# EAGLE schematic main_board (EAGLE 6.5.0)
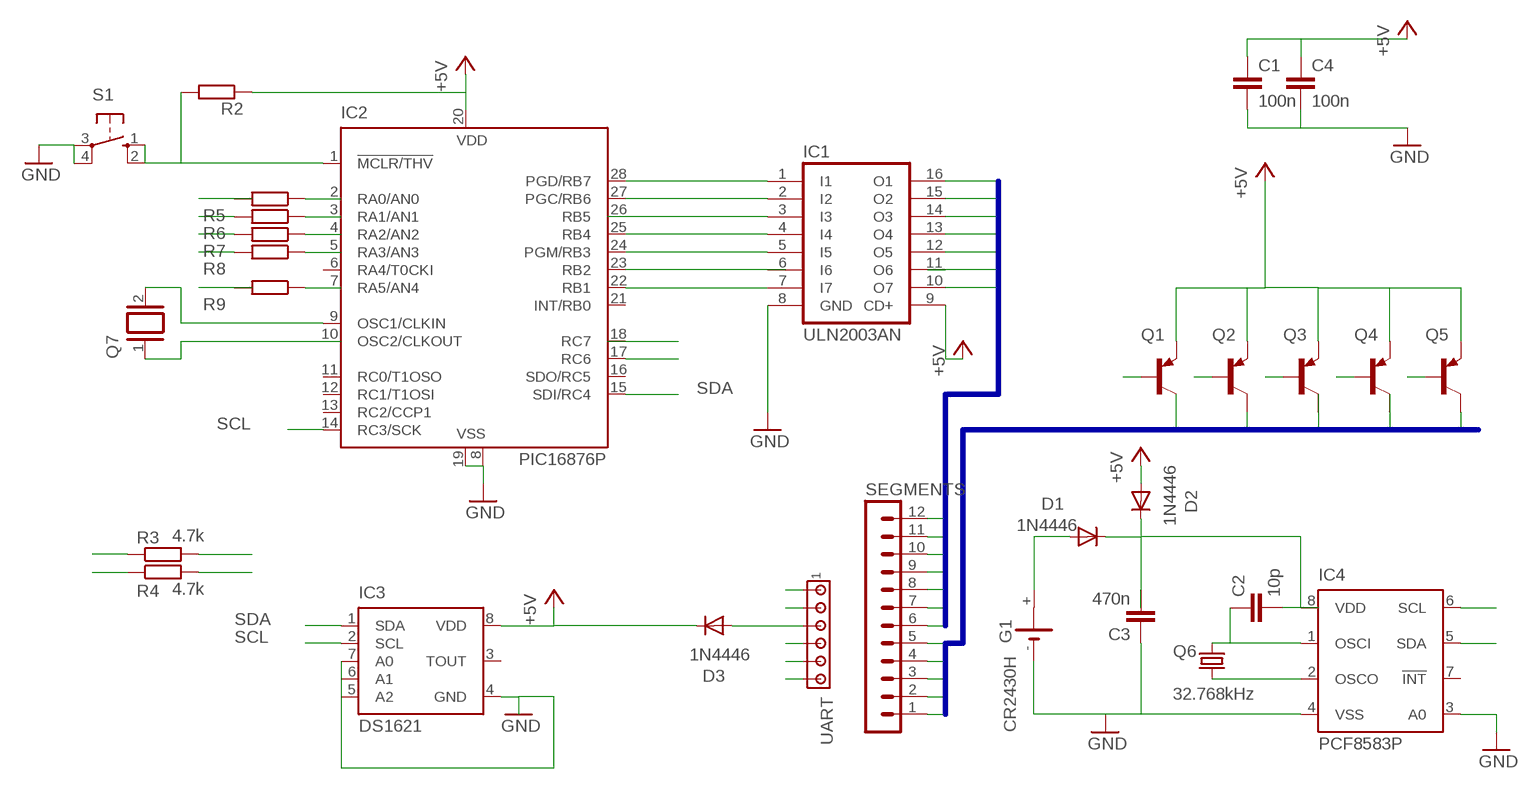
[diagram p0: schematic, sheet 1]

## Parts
C1  100n  C-EU025-030X050  [C025-030X050]
C2  10p  C-EU025-030X050  [C025-030X050]
C3  470n  C-EU025-030X050  [C025-030X050]
C4  100n  C-EU025-030X050  [C025-030X050]
D1  1N4446  [DO35-10]
D2  1N4446  [DO35-10]
D3  1N4446  [DO35-10]
G1  CR2430H  [CR2430H]
IC1  ULN2003AN  [DIL16]
IC2  PIC16876P  [DIL28-3]
IC3  DS1621  [DIL08]
IC4  PCF8583P  [DIL08]
Q1  BC369  [TO92-BCE]
Q2  BC369  [TO92-BCE]
Q3  BC369  [TO92-BCE]
Q4  BC369  [TO92-BCE]
Q5  BC369  [TO92-BCE]
Q6  32.768kHz  TF322J32K7680  [TF32]
Q7  XTAL  [Q]
R2  R-EU_0204/7  [0204/7]
R3  4.7k  R-EU_0204/7  [0204/7]
R4  4.7k  R-EU_0204/7  [0204/7]
R5  R-EU_0204/7  [0204/7]
R6  R-EU_0204/7  [0204/7]
R7  R-EU_0204/7  [0204/7]
R8  R-EU_0204/7  [0204/7]
R9  R-EU_0204/7  [0204/7]
S1  10-XX  [B3F-10XX]
SEGMENTS  MA12-1  [MA12-1]
UART  MTA06-100  [10X06MTA]

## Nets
+5V: C1.1 C4.1 D2.A D3.C IC1.9(CD+) IC2.20(VDD) IC3.8(VDD) Q1.E Q2.E Q3.E Q4.E Q5.E R3.1 R4.1
GND: C1.2 C3.1 C4.2 G1.- IC1.8(GND) IC2.8(VSS) IC2.19(VSS) IC4.3(A0) IC4.4(VSS) S1.3(P) S1.4(P1) UART.6
J_SEG_DATA0: IC1.16(O1) SEGMENTS.12
J_SEG_DATA1: IC1.15(O2) SEGMENTS.11
J_SEG_DATA2: IC1.14(O3) SEGMENTS.10
J_SEG_DATA3: IC1.13(O4) SEGMENTS.9
J_SEG_DATA4: IC1.12(O5) SEGMENTS.8
J_SEG_DATA5: IC1.11(O6) SEGMENTS.7
J_SEG_DATA6: IC1.10(O7) SEGMENTS.6
J_SEG_SELECT0: SEGMENTS.5
J_SEG_SELECT1: Q2.C SEGMENTS.4
J_SEG_SELECT2: SEGMENTS.3
J_SEG_SELECT3: SEGMENTS.2
J_SEG_SELECT4: Q5.C SEGMENTS.1
N$1: IC1.1(I1) IC2.28(PGD/RB7)
N$2: IC1.2(I2) IC2.27(PGC/RB6)
N$3: IC1.3(I3)
N$4: IC1.4(I4) IC2.25(RB4)
N$5: IC1.5(I5) IC2.24(PGM/RB3)
N$6: C2.1 IC4.1(OSCI) Q6.1
N$7: IC1.7(I7) IC2.22(RB1)
N$8: IC2.1(!MCLR/THV) R2.2 S1.1(S) S1.2(S1)
N$10: Q7.1
N$11: IC4.2(OSCO) Q6.2
N$12: D1.A G1.+
N$13: IC2.23(RB2)
N$14: IC3.4(GND) IC3.5(A2) IC3.6(A1) IC3.7(A0)
N$15: C2.2 C3.2 D1.C D2.C IC4.8(VDD)
N$16: IC2.9(OSC1/CLKIN) Q7.2
N$19: R9.1
N$20: R8.1
N$21: R7.1
N$22: R6.1
N$23: R5.1
N$24: R2.1
N$25: UART.5
N$26: D3.A UART.4
N$29: UART.1
SCL: IC2.14(RC3/SCK) IC3.2(SCL) IC4.6(SCL) R4.2
SDA: IC2.15(SDI/RC4) IC3.1(SDA) IC4.5(SDA) R3.2
SEG1: Q1.B
SEG2: Q2.B R6.2
SEG3: Q3.B R7.2
SEG4: Q4.B R8.2
SEG5: Q5.B
UART_RX: UART.3
UART_TX: IC2.17(RC6) UART.2
Unconnected: G1.+@1(+) IC1.6(I6) IC2.2(RA0/AN0) IC2.3(RA1/AN1) IC2.4(RA2/AN2) IC2.5(RA3/AN3) IC2.6(RA4/T0CKI) IC2.7(RA5/AN4) IC2.10(OSC2/CLKOUT) IC2.11(RC0/T1OSO) IC2.12(RC1/T1OSI) IC2.13(RC2/CCP1) IC2.16(SDO/RC5) IC2.18(RC7) IC2.21(INT/RB0) IC2.26(RB5) IC3.3(TOUT) IC4.7(!INT) Q1.C Q3.C Q4.C R5.2 R9.2

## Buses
J_SEG_DATA[0..6]
J_SEG_SELECT[0..4]

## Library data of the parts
C1-C4 = rcl:C-EU: CAPACITOR, European symbol
D1-D3 = diode:1N4446: DIODE
G1 = battery:CR2430H: LI BATTERY Varta
IC1 = uln-udn:ULN2003A: DRIVER ARRAY
IC2 = microchip:PIC16*876: MICROCONTROLLER flash type; OC_FARNELL: unknown; OC_NEWARK: unknown
IC3 = maxim:DS1621: Digital Thermometer and Thermostat Source: http://pdfserv.maxim-ic.com/en/ds/DS1621.pdf; MPN: DS1621; OC_FARNELL: 1188024; OC_NEWARK: 66F3769
IC4 = ds1307_pcf8583:PCF8583: I2C-Bus CLOCK/CALENDAR
Q1-Q5 = transistor-pnp:BC369*: PNP Transistror
Q6 = tf32:TF32: TF32 Series Tuning Fork Crystal; MF: CTS; MPN: TF322J32K7680; OC_FARNELL: unknown; OC_NEWARK: unknown
Q7 = special:XTAL: CRYSTAL
R2-R9 = rcl:R-EU_: RESISTOR, European symbol
S1 = switch-omron:10-XX: OMRON SWITCH; MPN: B3F-1000; OC_FARNELL: 176432; OC_NEWARK: 36M3542
SEGMENTS = con-lstb:MA12-1: PIN HEADER; OC_FARNELL: unknown; OC_NEWARK: unknown
UART = con-amp:MTA06-100: AMP connector

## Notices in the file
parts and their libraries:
tf32: (c) 2014 Samuel Lourenço
